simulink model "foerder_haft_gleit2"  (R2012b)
settings: Solver=ode2  StartTime=0.0  StopTime=10.0  FixedStep=dt  MaxStep=dt  RelTol=1e-3
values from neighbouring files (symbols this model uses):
  g = 9.89    [foerd_gleit_1.m]    (also in foerder_haft_gleit_1.m; foerder_haft_gleit_2.m; foerderband_1.m; position_reg_1.m)
  mu = m2/m1    (= 0.05)    [feder_masse_1.m]    (also in feder_masse_13.m; feder_masse_14.m; foerd_gleit_1.m = 0.9; foerder_haft_gleit_1.m = 0.5)

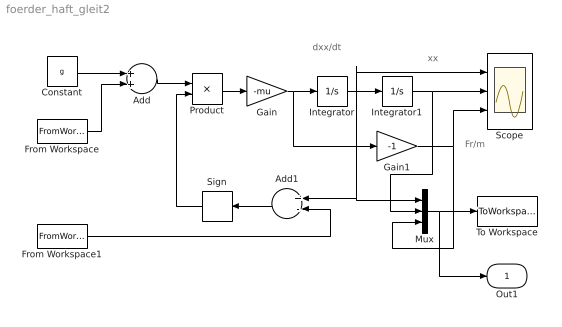
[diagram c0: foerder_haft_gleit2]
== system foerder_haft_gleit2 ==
  note: Fr/m
  note: xx
  note: dxx/dt
  Add : Sum
  Add1 : Sum  Inputs=+-
  Constant : Constant  Value=g
  From Workspace : FromWorkspace  VariableName=ay_m  SampleTime=0
  From Workspace1 : FromWorkspace  VariableName=vx_m  SampleTime=0
  Gain : Gain  Gain=-mu
  Gain1 : Gain  Gain=-1
  Integrator : Integrator
  Integrator1 : Integrator
  Mux : Mux  Inputs=3
  Product : Product
  Scope : Scope  NumInputPorts=3
  Sign : Signum  ZeroCross=off
  To Workspace : ToWorkspace  VariableName=y  SampleTime=-1  SaveFormat=Structure With Time
  Out1 : Outport
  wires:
  Constant/1 -> Add/1
  From Workspace/1 -> Add/2
  Product/1 -> Gain/1
  Integrator/1 -> Scope/1, Mux/1, Add1/1, Integrator1/1
  Sign/1 -> Product/2
  Add1/1 -> Sign/1
  Integrator1/1 -> Mux/2, Scope/2
  From Workspace1/1 -> Add1/2
  Add/1 -> Product/1
  Mux/1 -> Out1/1, To Workspace/1
  Gain/1 -> Gain1/1, Integrator/1
  Gain1/1 -> Mux/3, Scope/3
